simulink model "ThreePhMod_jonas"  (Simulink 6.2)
settings: Solver=ode23  StartTime=0  StopTime=0.02  FixedStep=0.000001  MaxStep=1e-5  RelTol=1e-3
undefined symbols (not defined in the file or in its folder): L, R, Sinus, Ts, Upp
libraries: simulink x3

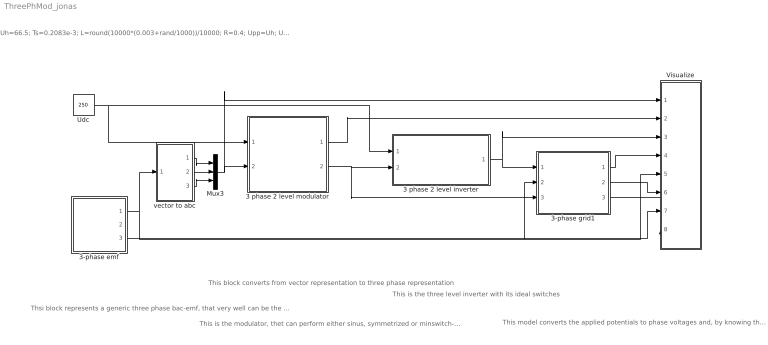
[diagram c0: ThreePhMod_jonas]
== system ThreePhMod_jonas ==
  note: Uh=66.5; Ts=0.2083e-3; L=round(10000*(0.003+rand/1000))/10000; R=0.4; Upp=Uh; Udc=250; Cdc=0.0011; di=3; Tf=1/(2*pi*30);
  note: Thsi block represents a generic three phase bac-emf, that very well can be the power line, having a 3-phase back-emf. In the same model, the back emf, the integral of the back emf (called "Psi") and the angle of the "Psi"- vetor is calculated. The three phase load model gives the output quantities in the alpha/beta reference frame, i.e. a vectors.
  note: This block converts from vector representation to three phase representation
  note: This is the modulator, thet can perform either sinus, symmetrized or minswitch- modulation with fixed or randomized carrier wave
  note: This is the three level inverter with its ideal switches
  note: This model converts the applied potentials to phase voltages and, by knowing the back-emf's it calculates the three phase currents. The phase voltages and phase currents are converted to vectors and serrved at the block output. The same block also calculates the DC link currents of the power electronic converter. This can be done if the switch positions and the phase currents are known. Hence, the switch position is supplied as input quantity.
  3 phase 2 level inverter : Subsystem
  3 phase 2 level modulator : Subsystem  mask{type=Sinus, Random=Fixed frequency, Ts=Ts}
      mask prompts: type "Sinus, Symmetrized or Minimum switch modulation"; Random "Fixed or random modulation?"; Ts "Sampling interval"
      mask help: Carrier Wave modulator that uses either fixed frequency modulation or random modulation. The fixed frequency modulation uses 1/(2Ts) as modulation frequency. The random modulation selects the modulatio frequency by random every sampling instant. The selection uses either 1/Ts, 1/(2Ts) or 1/(3Ts) as carrier wave frequency.
  3-phase emf : Subsystem  mask{Upp=Upp, freq=50, Tc=0.1e-3}
      mask prompts: Upp "U_phase_to_phase [RMS]"; freq "Frequency"; Tc "Sampling time"
  3-phase grid1 : Subsystem  mask{L=L, R=R}
      mask prompts: L "Inductance [H]"; R "Resistance [ohm]"
  Mux3 : Mux  Inputs=3
  Udc : Constant  Value=250
  Visualize : Subsystem
  vector to abc : Subsystem
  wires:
  Udc/1 -> 3 phase 2 level inverter/1(Udc), 3 phase 2 level modulator/1(Udc)
  3 phase 2 level modulator/2(sa,b,c) -> 3 phase 2 level inverter/2(sa,b,c), 3-phase grid1/3(s)
  3 phase 2 level modulator/1(mod) -> Visualize/2(mod)
  3 phase 2 level inverter/1(va,b,c) -> 3-phase grid1/1(va,b,c), Visualize/3(v)
  vector to abc/1(a) -> Mux3/1
  vector to abc/2(b) -> Mux3/2
  vector to abc/3(c) -> Mux3/3
  Mux3/1 -> 3 phase 2 level modulator/2(uabc*), Visualize/1(u*)
  3-phase emf/1(e_line) -> vector to abc/1(vect), 3-phase grid1/2(e_line), Visualize/5(e)
  3-phase grid1/1(u_ab) -> Visualize/4("u ")
  3-phase grid1/2(i_ab) -> Visualize/6(i)
  3-phase emf/3(Theta_line) -> Visualize/7(theta)
  3-phase grid1/3(i_dc) -> Visualize/8(idc)

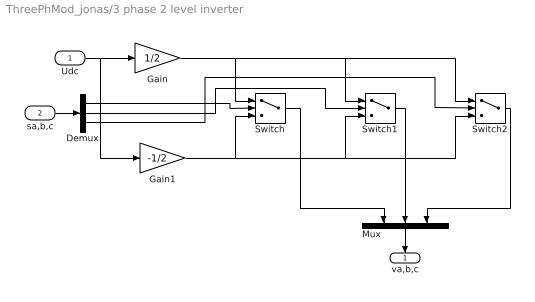
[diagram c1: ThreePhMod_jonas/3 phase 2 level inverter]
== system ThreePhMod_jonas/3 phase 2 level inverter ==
  Udc : Inport  Port=1  LatchInput=off
  sa,b,c : Inport  Port=2  LatchInput=off
  Demux : Demux  Outputs=3
  Gain : Gain  Gain=1/2
  Gain1 : Gain  Gain=-1/2
  Mux : Mux  Orientation=down  Inputs=3
  Switch : Switch
  Switch1 : Switch
  Switch2 : Switch
  va,b,c : Outport  Orientation=down  InitialOutput=0
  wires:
  Gain/1 -> Switch/1, Switch1/1, Switch2/1
  Gain1/1 -> Switch/3, Switch1/3, Switch2/3
  Udc/1 -> Gain1/1, Gain/1
  sa,b,c/1 -> Demux/1
  Demux/1 -> Switch/2
  Demux/2 -> Switch1/2
  Demux/3 -> Switch2/2
  Switch/1 -> Mux/1
  Switch1/1 -> Mux/2
  Switch2/1 -> Mux/3
  Mux/1 -> va,b,c/1

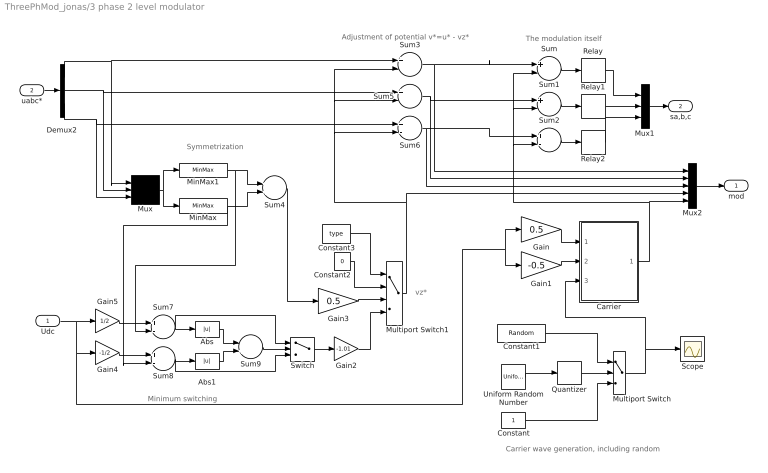
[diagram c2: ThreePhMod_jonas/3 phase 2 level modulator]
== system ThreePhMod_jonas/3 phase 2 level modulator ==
  note: Symmetrization
  note: vz*
  note: Minimum switching
  note: Adjustment of potential v*=u* - vz*
  note: The modulation itself
  note: Carrier wave generation, including random
  Udc : Inport  Port=1  LatchInput=off
  uabc* : Inport  Port=2  LatchInput=off
  Abs : Abs
  Abs1 : Abs
  Carrier : Subsystem
  Constant : Constant
  Constant1 : Constant  Value=Random
  Constant2 : Constant  Value=0
  Constant3 : Constant  Value=type
  Demux2 : Demux  Outputs=3
  Gain : Gain  Gain=0.5
  Gain1 : Gain  Gain=-0.5
  Gain2 : Gain  Gain=-1.01
  Gain3 : Gain  Gain=0.5
  Gain4 : Gain  Gain=-1/2
  Gain5 : Gain  Gain=1/2
  MinMax : MinMax
  MinMax1 : MinMax  Function=max
  Multiport Switch : MultiPortSwitch  Inputs=2
  Multiport Switch1 : MultiPortSwitch  Inputs=3
  Mux : Mux  Inputs=3
  Mux1 : Mux  Inputs=3
  Mux2 : Mux  Inputs=5
  Quantizer : Quantizer  QuantizationInterval=1
  Relay : Relay  OffOutputValue=-1
  Relay1 : Relay  OffOutputValue=-1
  Relay2 : Relay  OffOutputValue=-1
  Scope : Scope
  Sum{,1..3,5..8} (8 alike) : Sum  Inputs=+-
  Sum4 : Sum
  Sum9 : Sum  Inputs=-+
  Switch : Switch
  Uniform Random Number : UniformRandomNumber  Minimum=1  Maximum=3  Seed=0.9874  SampleTime=Ts
  mod : Outport  InitialOutput=0
  sa,b,c : Outport  Port=2  InitialOutput=0
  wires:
  Carrier/1(um) -> Sum2/2, Sum1/2, Sum/2, Mux2/5
  Gain1/1 -> Carrier/2(Umin)
  Gain/1 -> Carrier/1(Umax)
  Sum/1 -> Relay/1
  Relay1/1 -> Mux1/2
  Sum1/1 -> Relay1/1
  Relay2/1 -> Mux1/3
  Sum2/1 -> Relay2/1
  Sum3/1 -> Mux2/1, Sum/1
  Sum5/1 -> Mux2/2, Sum1/1
  Sum6/1 -> Mux2/3, Sum2/1
  Demux2/1 -> Sum3/1, Mux/1
  Demux2/2 -> Sum5/1, Mux/2
  Demux2/3 -> Sum6/1, Mux/3
  Mux/1 -> MinMax1/1, MinMax/1
  MinMax1/1 -> Sum4/1, Sum7/2
  MinMax/1 -> Sum4/2, Sum8/2
  Udc/1 -> Gain5/1, Gain4/1, Gain1/1, Gain/1
  Gain4/1 -> Sum8/1
  Sum7/1 -> Abs/1, Switch/1
  Sum8/1 -> Abs1/1, Switch/3
  Abs/1 -> Sum9/1
  Abs1/1 -> Sum9/2
  Sum9/1 -> Switch/2
  Sum4/1 -> Gain3/1
  Switch/1 -> Gain2/1
  Constant3/1 -> Multiport Switch1/1
  Constant2/1 -> Multiport Switch1/2
  Gain3/1 -> Multiport Switch1/3
  Gain2/1 -> Multiport Switch1/4
  Multiport Switch1/1 -> Sum5/2, Sum3/2, Sum6/2, Mux2/4
  Gain5/1 -> Sum7/1
  uabc*/1 -> Demux2/1
  Relay/1 -> Mux1/1
  Mux1/1 -> sa,b,c/1
  Mux2/1 -> mod/1
  Quantizer/1 -> Multiport Switch/2
  Uniform Random Number/1 -> Quantizer/1
  Constant/1 -> Multiport Switch/3
  Multiport Switch/1 -> Scope/1, Carrier/3(x)
  Constant1/1 -> Multiport Switch/1

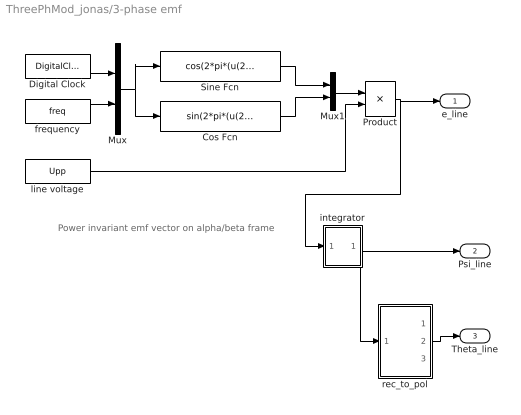
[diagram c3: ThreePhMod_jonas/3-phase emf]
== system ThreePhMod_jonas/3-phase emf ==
  note: Power invariant emf vector on alpha/beta frame
  Cos Fcn : Fcn  Expr=sin(2*pi*(u(2))*u(1)+pi/2)
  Digital Clock : DigitalClock  SampleTime=Tc
  Mux : Mux  Inputs=2
  Mux1 : Mux  Inputs=2
  Product : Product
  Sine Fcn : Fcn  Expr=cos(2*pi*(u(2))*u(1)+pi/2)
  frequency : Constant  Value=freq
  integrator : Subsystem
  line voltage : Constant  Value=Upp
  rec_to_pol : Subsystem
  e_line : Outport  InitialOutput=0
  Psi_line : Outport  Port=2  InitialOutput=0
  Theta_line : Outport  Port=3  InitialOutput=0
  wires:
  Product/1 -> e_line/1, integrator/1(In1)
  Mux1/1 -> Product/1
  Cos Fcn/1 -> Mux1/2
  Sine Fcn/1 -> Mux1/1
  Mux/1 -> Cos Fcn/1, Sine Fcn/1
  Digital Clock/1 -> Mux/1
  frequency/1 -> Mux/2
  line voltage/1 -> Product/2
  integrator/1(Out1) -> Psi_line/1, rec_to_pol/1(rect)
  rec_to_pol/2(angle) -> Theta_line/1

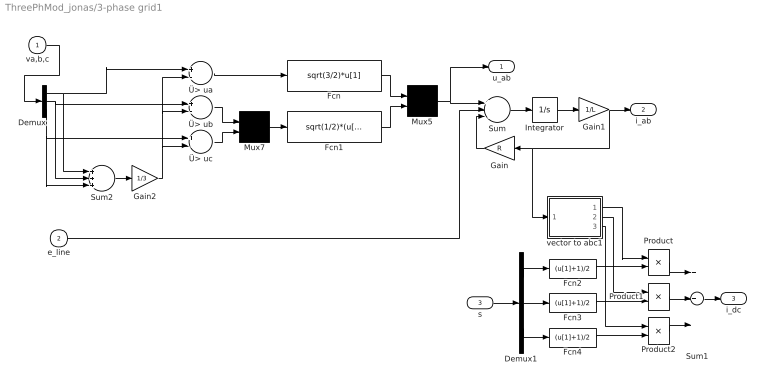
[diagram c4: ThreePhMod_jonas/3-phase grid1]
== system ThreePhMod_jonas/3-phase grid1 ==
  va,b,c : Inport  Port=1  LatchInput=off
  e_line : Inport  Port=2  LatchInput=off
  s : Inport  Port=3  LatchInput=off
  Demux : Demux  Outputs=3
  Demux1 : Demux  Outputs=3
  Fcn : Fcn  Expr=sqrt(3/2)*u[1]
  Fcn1 : Fcn  Expr=sqrt(1/2)*(u[1]-u[2])
  Fcn2 : Fcn  Expr=(u[1]+1)/2
  Fcn3 : Fcn  Expr=(u[1]+1)/2
  Fcn4 : Fcn  Expr=(u[1]+1)/2
  Gain : Gain  Orientation=left  Gain=R
  Gain1 : Gain  Gain=1/L
  Gain2 : Gain  Gain=1/3
  Integrator : Integrator
  Mux5 : Mux  Inputs=2
  Mux7 : Mux  Inputs=2
  Product : Product
  Product1 : Product
  Product2 : Product
  Sum : Sum  Inputs=+--
  Sum1 : Sum  Inputs=+++
  Sum2 : Sum  Inputs=+++
  vector to abc1 : Subsystem
  Ü> ua : Sum  Inputs=+-
  Ü> ub : Sum  Inputs=+-
  Ü> uc : Sum  Inputs=+-
  u_ab : Outport  InitialOutput=0
  i_ab : Outport  Port=2  InitialOutput=0
  i_dc : Outport  Port=3
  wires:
  Gain1/1 -> i_ab/1, Gain/1, vector to abc1/1(vect)
  Integrator/1 -> Gain1/1
  Gain/1 -> Sum/3
  Sum/1 -> Integrator/1
  Fcn1/1 -> Mux5/2
  Fcn/1 -> Mux5/1
  Mux5/1 -> Sum/1, u_ab/1
  Mux7/1 -> Fcn1/1
  Ü> uc/1 -> Mux7/2
  Ü> ub/1 -> Mux7/1
  Ü> ua/1 -> Fcn/1
  Gain2/1 -> Ü> uc/2, Ü> ub/2, Ü> ua/2
  Demux/2 -> Ü> ub/1, Sum2/2
  Sum2/1 -> Gain2/1
  Demux/3 -> Ü> uc/1, Sum2/3
  Demux/1 -> Ü> ua/1, Sum2/1
  va,b,c/1 -> Demux/1
  Demux1/2 -> Fcn3/1
  Demux1/1 -> Fcn2/1
  Demux1/3 -> Fcn4/1
  s/1 -> Demux1/1
  Sum1/1 -> i_dc/1
  Product2/1 -> Sum1/3
  Product1/1 -> Sum1/2
  Product/1 -> Sum1/1
  vector to abc1/1(a) -> Product/1
  vector to abc1/2(b) -> Product1/1
  vector to abc1/3(c) -> Product2/1
  Fcn4/1 -> Product2/2
  Fcn3/1 -> Product1/2
  Fcn2/1 -> Product/2
  e_line/1 -> Sum/2

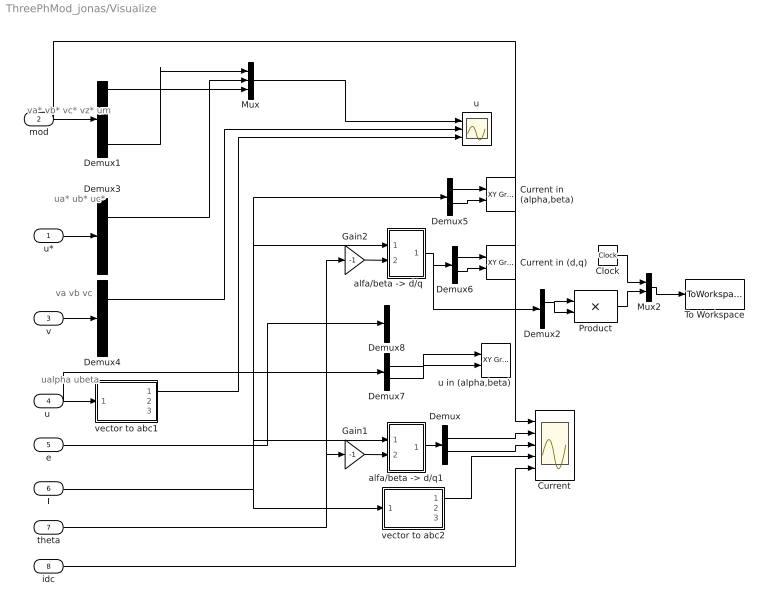
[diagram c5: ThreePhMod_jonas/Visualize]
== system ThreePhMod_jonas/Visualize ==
  note: va* vb* vc* vz* um
  note: ua* ub* uc*
  note: ualpha ubeta
  note: va vb vc
  u* : Inport  Port=1  LatchInput=off
  mod : Inport  Port=2  LatchInput=off
  v : Inport  Port=3  LatchInput=off
  "u " : Inport  Port=4  LatchInput=off
  e : Inport  Port=5  LatchInput=off
  i : Inport  Port=6  LatchInput=off
  theta : Inport  Port=7  LatchInput=off
  idc : Inport  Port=8  LatchInput=off
  Clock : Clock
  Current : Scope  NumInputPorts=5
  Current in (d,q) : simulink/Sinks/XY Graph  xmin=-5  xmax=5  ymin=-5  ymax=5  st=-1
  Current in  (alpha,beta) : simulink/Sinks/XY Graph  xmin=-5  xmax=5  ymin=-5  ymax=5  st=-1
  Demux{,2,5..8} (6 alike) : Demux  Outputs=2
  Demux1 : Demux  Outputs=5
  Demux3 : Demux  Outputs=3
  Demux4 : Demux  Outputs=3
  Gain1 : Gain  Gain=-1
  Gain2 : Gain  Gain=-1
  Mux : Mux  Inputs=3
  Mux2 : Mux  Inputs=2
  Product : Product
  To Workspace : ToWorkspace  VariableName=f1  SampleTime=-1  SaveFormat=Array
  "alfa/beta -> d/q" : Subsystem
  "alfa/beta -> d/q1" : Subsystem
  u : Scope  NumInputPorts=3
  u in (alpha,beta) : simulink/Sinks/XY Graph  xmin=-300  xmax=300  ymin=-300  ymax=300  st=-1
  vector to abc1 : Subsystem
  vector to abc2 : Subsystem
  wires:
  Gain2/1 -> "alfa/beta -> d/q"/2(angle)
  Gain1/1 -> "alfa/beta -> d/q1"/2(angle)
  "alfa/beta -> d/q1"/1(Out) -> Demux/1
  Demux/1 -> Current/2
  Demux/2 -> Current/3
  vector to abc2/1(a) -> Current/4
  mod/1 -> Demux1/1, Current/1
  "alfa/beta -> d/q"/1(Out) -> Demux2/1, Demux6/1
  Demux1/5 -> Mux/1
  Demux1/1 -> Mux/3
  Mux/1 -> u/1
  u*/1 -> Demux3/1
  "u "/1 -> vector to abc1/1(vect), Demux7/1
  Demux3/1 -> Mux/2
  v/1 -> Demux4/1
  Demux4/1 -> u/2
  vector to abc1/1(a) -> u/3
  i/1 -> "alfa/beta -> d/q"/1(vect), Demux5/1, "alfa/beta -> d/q1"/1(vect), vector to abc2/1(vect)
  e/1 -> Demux8/1
  theta/1 -> Gain1/1, Gain2/1
  Clock/1 -> Mux2/1
  Product/1 -> Mux2/2
  Mux2/1 -> To Workspace/1
  Demux2/1 -> Product/1, Product/2
  idc/1 -> Current/5
  Demux5/1 -> Current in  (alpha,beta)/1
  Demux5/2 -> Current in  (alpha,beta)/2
  Demux6/1 -> Current in (d,q)/1
  Demux6/2 -> Current in (d,q)/2
  Demux7/1 -> u in (alpha,beta)/1
  Demux7/2 -> u in (alpha,beta)/2

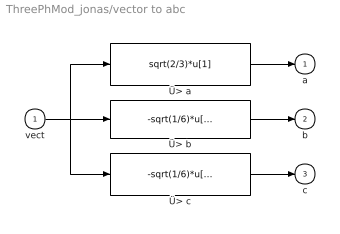
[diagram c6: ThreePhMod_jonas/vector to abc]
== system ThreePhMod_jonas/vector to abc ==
  vect : Inport  Port=1  LatchInput=off
  Ü> a : Fcn  Expr=sqrt(2/3)*u[1]
  Ü> b : Fcn  Expr=-sqrt(1/6)*u[1]+sqrt(1/2)*u[2]
  Ü> c : Fcn  Expr=-sqrt(1/6)*u[1]-sqrt(1/2)*u[2]
  a : Outport  InitialOutput=0
  b : Outport  Port=2  InitialOutput=0
  c : Outport  Port=3  InitialOutput=0
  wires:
  vect/1 -> Ü> b/1, Ü> a/1, Ü> c/1
  Ü> b/1 -> b/1
  Ü> c/1 -> c/1
  Ü> a/1 -> a/1

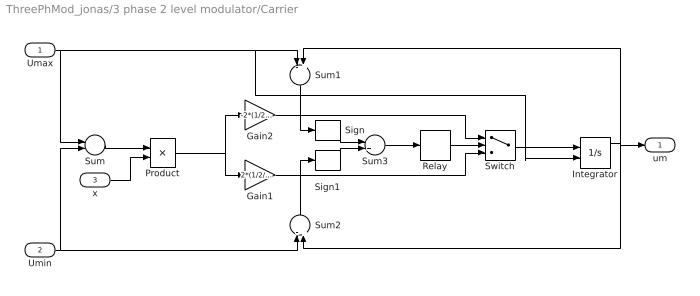
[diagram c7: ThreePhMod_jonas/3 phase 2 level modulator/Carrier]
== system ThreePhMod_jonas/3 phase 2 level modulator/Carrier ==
  Umax : Inport  Port=1  LatchInput=off
  Umin : Inport  Port=2  LatchInput=off
  x : Inport  Port=3  LatchInput=off
  Gain1 : Gain  Gain=2*(1/2/Ts)
  Gain2 : Gain  Gain=-2*(1/2/Ts)
  Integrator : Integrator  InitialConditionSource=external
  Product : Product
  Relay : Relay  OnSwitchValue=1  OffSwitchValue=-1  OffOutputValue=-1
  Sign : Signum
  Sign1 : Signum
  Sum : Sum  Inputs=+-
  Sum1 : Sum  Orientation=down  Inputs=-+
  Sum2 : Sum  Orientation=up  Inputs=-+
  Sum3 : Sum
  Switch : Switch
  um : Outport
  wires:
  Switch/1 -> Integrator/1
  Umax/1 -> Sum/1, Sum1/1, Integrator/2
  Umin/1 -> Sum/2, Sum2/1
  Gain2/1 -> Switch/1
  Gain1/1 -> Switch/3
  Integrator/1 -> Sum1/2, um/1, Sum2/2
  Sum1/1 -> Sign/1
  Sum2/1 -> Sign1/1
  Sign/1 -> Sum3/1
  Sign1/1 -> Sum3/2
  Sum3/1 -> Relay/1
  Relay/1 -> Switch/2
  Sum/1 -> Product/1
  Product/1 -> Gain2/1, Gain1/1
  x/1 -> Product/2

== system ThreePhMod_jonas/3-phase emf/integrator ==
  note: Power invariant emf vector on alpha/beta frame
  In1 : Inport  Port=1  LatchInput=off
  Demux : Demux  Outputs=2
  Integrator1 : Integrator  InitialCondition=Upp/(2*pi*freq)
  Integrator2 : Integrator
  Mux : Mux  Inputs=2
  Out1 : Outport
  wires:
  In1/1 -> Demux/1
  Mux/1 -> Out1/1
  Integrator2/1 -> Mux/2
  Integrator1/1 -> Mux/1
  Demux/2 -> Integrator2/1
  Demux/1 -> Integrator1/1

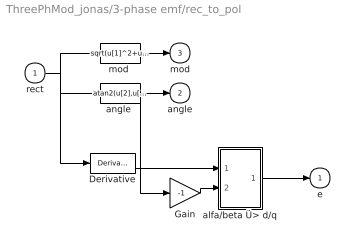
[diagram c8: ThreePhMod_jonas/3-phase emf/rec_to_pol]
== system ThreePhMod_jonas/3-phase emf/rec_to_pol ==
  rect : Inport  Port=1  LatchInput=off
  Derivative : Derivative
  Gain : Gain  Gain=-1
  alfa/beta Ü> d/q : Subsystem
  "angle " : Fcn  Expr=atan2(u[2],u[1])
  "mod " : Fcn  Expr=sqrt(u[1]^2+u[2]^2)
  e : Outport  InitialOutput=0
  angle : Outport  Port=2  InitialOutput=0
  mod : Outport  Port=3  InitialOutput=0
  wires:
  "angle "/1 -> angle/1, Gain/1
  rect/1 -> "angle "/1, "mod "/1, Derivative/1
  "mod "/1 -> mod/1
  Gain/1 -> alfa/beta Ü> d/q/2(angle)
  Derivative/1 -> alfa/beta Ü> d/q/1(vect)
  alfa/beta Ü> d/q/1(Out) -> e/1

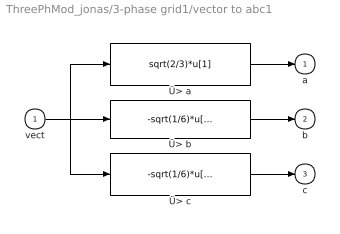
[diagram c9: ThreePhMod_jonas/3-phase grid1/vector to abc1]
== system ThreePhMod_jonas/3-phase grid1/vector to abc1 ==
  vect : Inport  Port=1  LatchInput=off
  Ü> a : Fcn  Expr=sqrt(2/3)*u[1]
  Ü> b : Fcn  Expr=-sqrt(1/6)*u[1]+sqrt(1/2)*u[2]
  Ü> c : Fcn  Expr=-sqrt(1/6)*u[1]-sqrt(1/2)*u[2]
  a : Outport  InitialOutput=0
  b : Outport  Port=2  InitialOutput=0
  c : Outport  Port=3  InitialOutput=0
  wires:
  vect/1 -> Ü> b/1, Ü> a/1, Ü> c/1
  Ü> b/1 -> b/1
  Ü> c/1 -> c/1
  Ü> a/1 -> a/1

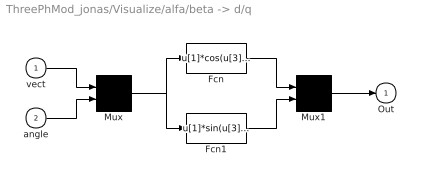
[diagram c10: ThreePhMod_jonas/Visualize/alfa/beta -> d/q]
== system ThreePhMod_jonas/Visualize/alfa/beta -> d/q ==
  vect : Inport  Port=1  LatchInput=off
  angle : Inport  Port=2  LatchInput=off
  Fcn : Fcn  Expr=u[1]*cos(u[3])-u[2]*sin(u[3])
  Fcn1 : Fcn  Expr=u[1]*sin(u[3])+u[2]*cos(u[3])
  Mux : Mux  Inputs=2
  Mux1 : Mux  Inputs=2
  Out : Outport  InitialOutput=0
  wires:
  vect/1 -> Mux/1
  angle/1 -> Mux/2
  Mux/1 -> Fcn/1, Fcn1/1
  Fcn/1 -> Mux1/1
  Fcn1/1 -> Mux1/2
  Mux1/1 -> Out/1

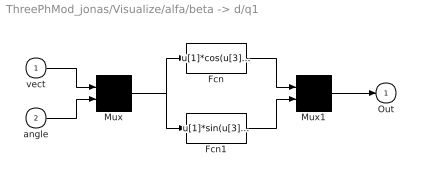
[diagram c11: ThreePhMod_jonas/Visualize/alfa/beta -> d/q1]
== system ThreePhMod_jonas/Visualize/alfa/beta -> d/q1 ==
  vect : Inport  Port=1  LatchInput=off
  angle : Inport  Port=2  LatchInput=off
  Fcn : Fcn  Expr=u[1]*cos(u[3])-u[2]*sin(u[3])
  Fcn1 : Fcn  Expr=u[1]*sin(u[3])+u[2]*cos(u[3])
  Mux : Mux  Inputs=2
  Mux1 : Mux  Inputs=2
  Out : Outport  InitialOutput=0
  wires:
  Mux1/1 -> Out/1
  Fcn1/1 -> Mux1/2
  Fcn/1 -> Mux1/1
  Mux/1 -> Fcn1/1, Fcn/1
  angle/1 -> Mux/2
  vect/1 -> Mux/1

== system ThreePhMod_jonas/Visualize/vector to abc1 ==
  vect : Inport  Port=1  LatchInput=off
  Ü> a : Fcn  Expr=sqrt(2/3)*u[1]
  Ü> b : Fcn  Expr=-sqrt(1/6)*u[1]+sqrt(1/2)*u[2]
  Ü> c : Fcn  Expr=-sqrt(1/6)*u[1]-sqrt(1/2)*u[2]
  a : Outport  InitialOutput=0
  b : Outport  Port=2  InitialOutput=0
  c : Outport  Port=3  InitialOutput=0
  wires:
  Ü> a/1 -> a/1
  Ü> c/1 -> c/1
  Ü> b/1 -> b/1
  vect/1 -> Ü> c/1, Ü> a/1, Ü> b/1

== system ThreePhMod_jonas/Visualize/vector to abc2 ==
  vect : Inport  Port=1  LatchInput=off
  Ü> a : Fcn  Expr=sqrt(2/3)*u[1]
  Ü> b : Fcn  Expr=-sqrt(1/6)*u[1]+sqrt(1/2)*u[2]
  Ü> c : Fcn  Expr=-sqrt(1/6)*u[1]-sqrt(1/2)*u[2]
  a : Outport  InitialOutput=0
  b : Outport  Port=2  InitialOutput=0
  c : Outport  Port=3  InitialOutput=0
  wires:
  vect/1 -> Ü> b/1, Ü> a/1, Ü> c/1
  Ü> b/1 -> b/1
  Ü> c/1 -> c/1
  Ü> a/1 -> a/1

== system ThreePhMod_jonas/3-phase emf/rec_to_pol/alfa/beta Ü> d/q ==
  vect : Inport  Port=1  LatchInput=off
  angle : Inport  Port=2  LatchInput=off
  Fcn : Fcn  Expr=u[1]*cos(u[3])-u[2]*sin(u[3])
  Fcn1 : Fcn  Expr=u[1]*sin(u[3])+u[2]*cos(u[3])
  Mux : Mux  Inputs=2
  Mux1 : Mux  Inputs=2
  Out : Outport  InitialOutput=0
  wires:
  vect/1 -> Mux/1
  angle/1 -> Mux/2
  Mux/1 -> Fcn/1, Fcn1/1
  Fcn/1 -> Mux1/1
  Fcn1/1 -> Mux1/2
  Mux1/1 -> Out/1
